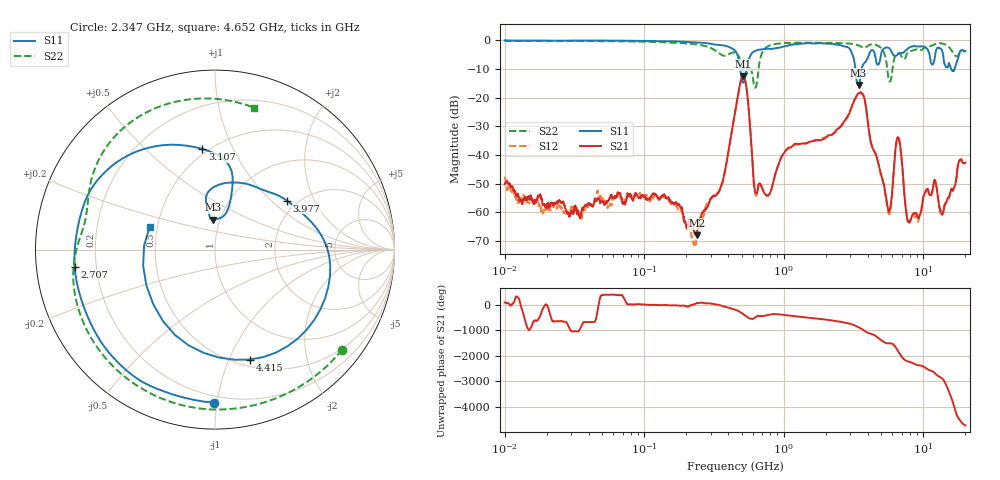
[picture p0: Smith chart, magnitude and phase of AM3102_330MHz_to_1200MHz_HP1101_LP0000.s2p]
! Date/Time: Tue, Sep 11, 2018 5:21 PM
! Network Analyzer: Agilent Technologies E8362B Rev: A.07.50.63
! Sweep from 0.010 to 20.000 GHz, 1601 Points, Sweep Type: LOG
! Power Supply: 4.949 V, 0.001 A
# Hz S DB R 50
!freq MagS11 AngS11 MagS21 AngS21 MagS12 AngS12 MagS22 AngS22
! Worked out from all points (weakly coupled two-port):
!   1601 points, 10 MHz to 20 GHz, reference 50 ohm
!   highest |S21| = -12.60 dB at 510.8 MHz (marker M1); lowest = -68.1 dB at 237.7 MHz (marker M2)
!   lowest |S11| = -15.6 dB at 3.432 GHz (marker M3), VSWR 1.40, Z = 46.3 + j15.8 ohm
!   |S11| at or under -10 dB: 486.3 MHz to 541.7 MHz (55.37 MHz wide, 10.8 % of centre); 3.25 GHz to 3.604 GHz (353 MHz wide, 10.3 % of centre); 15.86 GHz to 16.73 GHz (872.6 MHz wide, 5.35 % of centre)
!   |S22| runs from -16.5 to -0.2 dB; largest |S21 - S12| = 0.0057
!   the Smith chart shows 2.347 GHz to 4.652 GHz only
!   S11 on the Smith chart (normalised r, x): 2.347 GHz: 0.16, -0.98; 2.707 GHz: 0.12, -0.06; 3.107 GHz: 0.47, +0.77; 3.977 GHz: 1.77, +1.26; 4.415 GHz: 0.57, -1.19; 4.652 GHz: 0.45, +0.14
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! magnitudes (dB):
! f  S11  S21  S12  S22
! 10 MHz  0.0  -50.3  -47.6  -0.2
! 35.55 MHz  -0.1  -59.5  -62.1  -0.2
! 126.4 MHz  -0.2  -55.2  -55.4  -0.6
! 237.7 MHz  -0.7  -68.1  -69.7  -1.4
! 357.7 MHz  -1.7  -50.6  -50.9  -5.1
! 447.2 MHz  -3.5  -25.1  -25.2  -4.3
! 510.8 MHz  -14.8  -12.6  -12.6  -11.0
! 632.6 MHz  -3.6  -53.5  -54.2  -16.2
! 757.7 MHz  -2.9  -54.1  -54.3  -2.3
! 1.59 GHz  -1.0  -35.2  -35.2  -0.8
! 2.347 GHz  -1.4  -31.7  -32.1  -0.9
! 2.707 GHz  -2.1  -28.2  -28.6  -1.0
! 3.107 GHz  -4.9  -22.3  -22.5  -1.2
! 3.432 GHz  -15.6  -18.5  -18.6  -1.8
! 3.977 GHz  -6.3  -27.5  -27.3  -2.0
! 4.415 GHz  -3.8  -38.5  -38.4  -1.4
! 4.652 GHz  -8.3  -41.0  -41.1  -1.7
! 5.652 GHz  -2.6  -59.7  -60.7  -13.7
! 6.549 GHz  -4.9  -33.8  -34.1  -4.6
! 7.92 GHz  -2.5  -63.6  -63.1  -3.9
! 13.68 GHz  -3.9  -60.9  -59.6  -1.1
! 20 GHz  -3.8  -42.7  -43.2  -3.8
